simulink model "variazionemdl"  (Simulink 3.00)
settings: Solver=ode45  StartTime=0.0  StopTime=10.0  RelTol=1e-3
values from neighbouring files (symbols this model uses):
  d0 = 0;0.5    [variazione.m]
  k = tau0/tau1 -1    (= 39)    [variazione.m]
  r0 = 1    [variazione.m]
  tau = 0.5*tau0    (= 20)    [variazione.m]
  tau0 = 40    [variazione.m]
  tau1 = 1    [variazione.m]

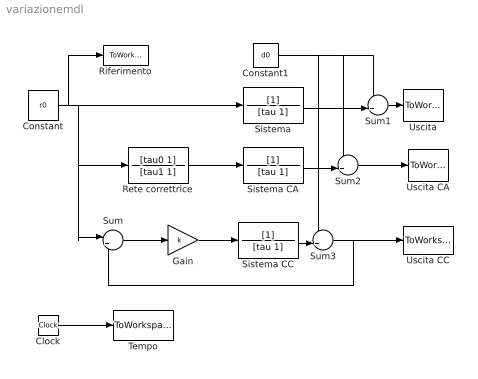
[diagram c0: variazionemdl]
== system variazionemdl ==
  Clock : Clock
  Constant : Constant  Value=r0
  Constant1 : Constant  Value=d0
  Gain : Gain  Gain=k  SaturateOnIntegerOverflow=on
  Rete correttrice : TransferFcn  Numerator=[tau0 1]  Denominator=[tau1 1]
  Riferimento : ToWorkspace  VariableName=r  SampleTime=-1  SaveFormat=Matrix
  Sistema : TransferFcn  Numerator=[1]  Denominator=[tau 1]
  Sistema CA : TransferFcn  Numerator=[1]  Denominator=[tau 1]
  Sistema CC : TransferFcn  Numerator=[1]  Denominator=[tau 1]
  Sum : Sum  Inputs=|+-  SaturateOnIntegerOverflow=on
  Sum1 : Sum  Inputs=++|  SaturateOnIntegerOverflow=on
  Sum2 : Sum  Inputs=++|  SaturateOnIntegerOverflow=on
  Sum3 : Sum  Inputs=++|  SaturateOnIntegerOverflow=on
  Tempo : ToWorkspace  VariableName=t  SampleTime=-1  SaveFormat=Matrix
  Uscita : ToWorkspace  VariableName=y  SampleTime=-1  SaveFormat=Matrix
  Uscita CA : ToWorkspace  VariableName=yca  SampleTime=-1  SaveFormat=Matrix
  Uscita CC : ToWorkspace  VariableName=ycc  SampleTime=-1  SaveFormat=Matrix
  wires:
  Constant/1 -> Riferimento/1, Sistema/1, Sum/1, Rete correttrice/1
  Clock/1 -> Tempo/1
  Gain/1 -> Sistema CC/1
  Sum/1 -> Gain/1
  Rete correttrice/1 -> Sistema CA/1
  Sistema/1 -> Sum1/2
  Sistema CA/1 -> Sum2/2
  Sistema CC/1 -> Sum3/2
  Sum1/1 -> Uscita/1
  Sum2/1 -> Uscita CA/1
  Sum3/1 -> Uscita CC/1, Sum/2
  Constant1/1 -> Sum1/1, Sum2/1, Sum3/1
